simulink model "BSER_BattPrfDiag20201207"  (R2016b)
settings: Solver=FixedStepDiscrete  StartTime=0.0  StopTime=10.0  FixedStep=0.02  RelTol=1e-3  EnableMultiTasking=on
undefined symbols (not defined in the file or in its folder): bin2dec, BSER_cntBattOCMinDiag_C, BSER_cntBattPrfDiag_CW, BSER_cntChrgOCNpl_C, BSER_cntDisChOCNpl_C, BSER_cntPwrConvertConst_C, BSER_iChrgCurrErr_C, BSER_iChrgCurrOk_C, BSER_iDisChCurrErr_C, BSER_iDisChCurrOk_C, BSER_iLonChrgCurrErr_C, BSER_iLonChrgCurrOk_C, BSER_iLonDisChCurrErr_C, BSER_iLonDisChCurrOk_C, BSER_iShrtChrgCurrErr_C, BSER_iShrtChrgCurrOk_C, BSER_iShrtDisChCurrErr_C, BSER_iShrtDisChCurrOk_C, BSER_iSumLonChrgCurrReq_C, BSER_iSumLonDisChCurrReq_C, BSER_iSumShrtChrgCurrReq_C, BSER_iSumShrtDisChCurrReq_C, BSER_rLonChrgCurrHeal_C, BSER_rLonChrgCurrHi_C, BSER_rLonDisChCurrHeal_C, BSER_rLonDisChCurrHi_C, BSER_rShrtChrgCurrHeal_C, BSER_rShrtChrgCurrHi_C, BSER_rShrtDisChCurrHeal_C, BSER_rShrtDisChCurrHi_C, BSER_tiChrgCurrErr_C, BSER_tiChrgCurrOk_C, BSER_tiCurrConstPer_C, BSER_tiCurrPeakPer_C, BSER_tiDisChCurrErr_C, BSER_tiDisChCurrOk_C, BSER_uBattVoltConst_C
libraries: simulink x68
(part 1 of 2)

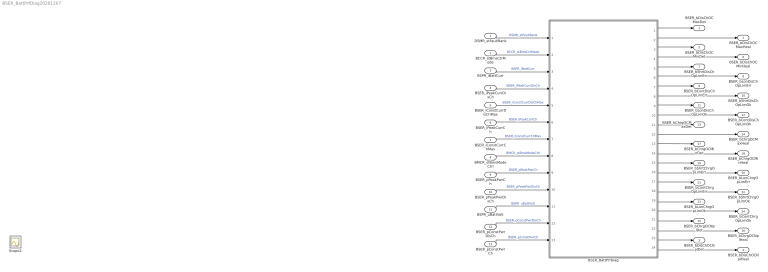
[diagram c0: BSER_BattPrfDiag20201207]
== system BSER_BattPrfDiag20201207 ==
  DSMR_stFaultRank : Inport
  BCCR_stBmsCtrMode : Inport  Port=2
  BSPR_iBattCurr : Inport  Port=3
  BSER_iPeakCurrDisCh : Inport  Port=4
  BSER_iConstCurrDisChMax : Inport  Port=5
  BSER_iPeakCurrCh : Inport  Port=6
  BSER_iConstCurrChMax : Inport  Port=7
  BMCR_stBmsModeCtrl : Inport  Port=8
  BSER_pPeakPwrCh : Inport  Port=9
  BSER_pPeakPwrDisCh : Inport  Port=10
  BSPR_uBattVolt : Inport  Port=11
  BSER_pConstPwrDisCh : Inport  Port=12
  BSER_pConstPwrCh : Inport  Port=13
  BSER_BattPrfDiag : Subsystem
  BSER_bDisChOCMaxDet : Outport
  BSER_bDisChOCMaxHeal : Outport  Port=2
  BSER_bDisChOCNplDet : Outport  Port=3
  BSER_bDisChOCNplHeal : Outport  Port=4
  BSER_bDisChOCMinDet : Outport  Port=5
  BSER_bDisChOCMinHeal : Outport  Port=6
  BSER_bShrtDisChOpLimErr : Outport  Port=7
  BSER_bLonDisChOpLimErr : Outport  Port=8
  BSER_bContDisChOpLimErr : Outport  Port=9
  BSER_bShrtDisChOpLimOk : Outport  Port=10
  BSER_bLonDisChOpLimOk : Outport  Port=11
  BSER_bContDisChOpLimOk : Outport  Port=12
  BSER_bChrgOCMaxDet : Outport  Port=13
  BSER_bChrgOCMaxHeal : Outport  Port=14
  BSER_bChrgOCNplDet : Outport  Port=15
  BSER_bChrgOCNplHeal : Outport  Port=16
  BSER_bChrgOCMinDet : Outport  Port=17
  BSER_bChrgOCMinHeal : Outport  Port=18
  BSER_bShrtChrgOpLimErr : Outport  Port=19
  BSER_bLonChrgOpLimErr : Outport  Port=20
  BSER_bContChrgOpLimErr : Outport  Port=21
  BSER_bShrtChrgOpLimOk : Outport  Port=22
  BSER_bLonChrgOpLimOk : Outport  Port=23
  BSER_bContChrgOpLimOk : Outport  Port=24
  Scope2 : Scope
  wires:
  DSMR_stFaultRank/1 -> BSER_BattPrfDiag/1(DSMR_stFaultRank)  "DSMR_stFaultRank"
  BCCR_stBmsCtrMode/1 -> BSER_BattPrfDiag/2(BCCR_stBmsCtrMode)  "BCCR_stBmsCtrMode"
  BSPR_iBattCurr/1 -> BSER_BattPrfDiag/3(BSPR_iBattCurr)  "BSPR_iBattCurr"
  BSER_iPeakCurrDisCh/1 -> BSER_BattPrfDiag/4(BSER_iPeakCurrDisCh)  "BSER_iPeakCurrDisCh"
  BSER_iConstCurrDisChMax/1 -> BSER_BattPrfDiag/5(BSER_iConstCurrDisChMax)  "BSER_iConstCurrDisChMax"
  BSER_iPeakCurrCh/1 -> BSER_BattPrfDiag/6(BSER_iPeakCurrCh)  "BSER_iPeakCurrCh"
  BSER_iConstCurrChMax/1 -> BSER_BattPrfDiag/7(BSER_iConstCurrChMax)  "BSER_iConstCurrChMax"
  BSER_BattPrfDiag/1(BSER_bDisChOCMaxDet) -> BSER_bDisChOCMaxDet/1
  BSER_BattPrfDiag/2(BSER_bDisChOCMaxHeal) -> BSER_bDisChOCMaxHeal/1
  BSER_BattPrfDiag/3(BSER_bDisChOCMinDet) -> BSER_bDisChOCMinDet/1
  BSER_BattPrfDiag/4(BSER_bDisChOCMinHeal) -> BSER_bDisChOCMinHeal/1
  BSER_BattPrfDiag/5(BSER_bShrtDisChOpLimErr) -> BSER_bShrtDisChOpLimErr/1
  BSER_BattPrfDiag/6(BSER_bLonDisChOpLimErr) -> BSER_bLonDisChOpLimErr/1
  BSER_BattPrfDiag/7(BSER_bContDisChOpLimErr) -> BSER_bContDisChOpLimErr/1
  BSER_BattPrfDiag/8(BSER_bShrtDisChOpLimOk) -> BSER_bShrtDisChOpLimOk/1
  BSER_BattPrfDiag/9(BSER_bLonDisChOpLimOk) -> BSER_bLonDisChOpLimOk/1
  BSER_BattPrfDiag/10(BSER_bContDisChOpLimOk) -> BSER_bContDisChOpLimOk/1
  BSER_BattPrfDiag/11(BSER_bChrgOCMaxDet) -> BSER_bChrgOCMaxDet/1
  BSER_BattPrfDiag/12(BSER_bChrgOCMaxHeal) -> BSER_bChrgOCMaxHeal/1
  BSER_BattPrfDiag/13(BSER_bChrgOCMinDet) -> BSER_bChrgOCMinDet/1
  BSER_BattPrfDiag/14(BSER_bChrgOCMinHeal) -> BSER_bChrgOCMinHeal/1
  BSER_BattPrfDiag/15(BSER_bShrtChrgOpLimErr) -> BSER_bShrtChrgOpLimErr/1
  BSER_BattPrfDiag/16(BSER_bLonChrgOpLimErr) -> BSER_bLonChrgOpLimErr/1
  BSER_BattPrfDiag/17(BSER_bContChrgOpLimErr) -> BSER_bContChrgOpLimErr/1
  BSER_BattPrfDiag/18(BSER_bShrtChrgOpLimOk) -> BSER_bShrtChrgOpLimOk/1
  BSER_BattPrfDiag/19(BSER_bLonChrgOpLimOk) -> BSER_bLonChrgOpLimOk/1
  BSER_BattPrfDiag/20(BSER_bContChrgOpLimOk) -> BSER_bContChrgOpLimOk/1
  BSER_BattPrfDiag/23(BSER_bDisChOCNplDet) -> BSER_bDisChOCNplDet/1
  BSER_BattPrfDiag/24(BSER_bDisChOCNplHeal) -> BSER_bDisChOCNplHeal/1
  BSER_BattPrfDiag/21(BSER_bChrgOCNplDet) -> BSER_bChrgOCNplDet/1
  BSER_BattPrfDiag/22(BSER_bChrgOCNplHeal) -> BSER_bChrgOCNplHeal/1
  BMCR_stBmsModeCtrl/1 -> BSER_BattPrfDiag/8(BMCR_stBmsModeCtrl)  "BMCR_stBmsModeCtrl"
  BSER_pPeakPwrDisCh/1 -> BSER_BattPrfDiag/10(BSER_pPeakPwrDisCh)  "BSER_pPeakPwrDisCh"
  BSER_pPeakPwrCh/1 -> BSER_BattPrfDiag/9(BSER_pPeakPwrCh)  "BSER_pPeakPwrCh"
  BSPR_uBattVolt/1 -> BSER_BattPrfDiag/11(BSPR_uBattVolt)  "BSPR_uBattVolt"
  BSER_pConstPwrCh/1 -> BSER_BattPrfDiag/13(BSER_pConstPwrCh)  "BSER_pConstPwrCh"
  BSER_pConstPwrDisCh/1 -> BSER_BattPrfDiag/12(BSER_pConstPwrDisCh)  "BSER_pConstPwrDisCh"

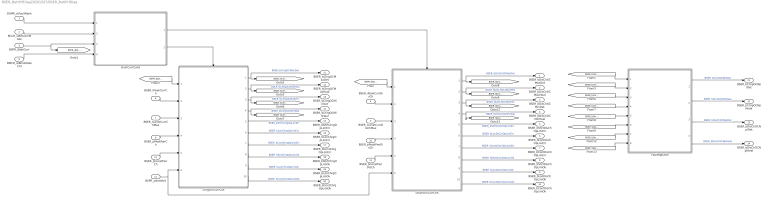
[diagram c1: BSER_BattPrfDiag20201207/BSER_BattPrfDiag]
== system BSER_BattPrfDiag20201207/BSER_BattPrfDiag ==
  DSMR_stFaultRank : Inport
  BCCR_stBmsCtrMode : Inport  Port=2
  BSPR_iBattCurr : Inport  Port=3
  BSER_iPeakCurrDisCh : Inport  Port=4
  BSER_iConstCurrDisChMax : Inport  Port=5
  BSER_iPeakCurrCh : Inport  Port=6
  BSER_iConstCurrChMax : Inport  Port=7
  BMCR_stBmsModeCtrl : Inport  Port=8
  BSER_pPeakPwrCh : Inport  Port=9
  BSER_pPeakPwrDisCh : Inport  Port=10
  BSPR_uBattVolt : Inport  Port=11
  BSER_pConstPwrDisCh : Inport  Port=12
  BSER_pConstPwrCh : Inport  Port=13
  ChrgOvrCurrChk : Subsystem
  DischOvrCurrChk : Subsystem
  FaultRptDsm : Subsystem
  OverCurrCond : Subsystem
  BSER_bDisChOCMaxDet : Outport
  BSER_bDisChOCMaxHeal : Outport  Port=2
  BSER_bDisChOCMinDet : Outport  Port=3
  BSER_bDisChOCMinHeal : Outport  Port=4
  BSER_bShrtDisChOpLimErr : Outport  Port=5
  BSER_bLonDisChOpLimErr : Outport  Port=6
  BSER_bContDisChOpLimErr : Outport  Port=7
  BSER_bShrtDisChOpLimOk : Outport  Port=8
  BSER_bLonDisChOpLimOk : Outport  Port=9
  BSER_bContDisChOpLimOk : Outport  Port=10
  BSER_bChrgOCMaxDet : Outport  Port=11
  BSER_bChrgOCMaxHeal : Outport  Port=12
  BSER_bChrgOCMinDet : Outport  Port=13
  BSER_bChrgOCMinHeal : Outport  Port=14
  BSER_bShrtChrgOpLimErr : Outport  Port=15
  BSER_bLonChrgOpLimErr : Outport  Port=16
  BSER_bContChrgOpLimErr : Outport  Port=17
  BSER_bShrtChrgOpLimOk : Outport  Port=18
  BSER_bLonChrgOpLimOk : Outport  Port=19
  BSER_bContChrgOpLimOk : Outport  Port=20
  BSER_bChrgOCNplDet : Outport  Port=21
  BSER_bChrgOCNplHeal : Outport  Port=22
  BSER_bDisChOCNplDet : Outport  Port=23
  BSER_bDisChOCNplHeal : Outport  Port=24
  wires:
  ChrgOvrCurrChk/10(BSER_bContChrgOpLimOk) -> BSER_bContChrgOpLimOk/1  "BSER_bContChrgOpLimOk"
  ChrgOvrCurrChk/9(BSER_bLonChrgOpLimOk) -> BSER_bLonChrgOpLimOk/1  "BSER_bLonChrgOpLimOk"
  ChrgOvrCurrChk/8(BSER_bShrtChrgOpLimOk) -> BSER_bShrtChrgOpLimOk/1  "BSER_bShrtChrgOpLimOk"
  ChrgOvrCurrChk/7(BSER_bContChrgOpLimErr) -> BSER_bContChrgOpLimErr/1  "BSER_bContChrgOpLimErr"
  ChrgOvrCurrChk/3(BSER_bChrgOCMinDet) -> [BSER_bChrgOCMinDet], BSER_bChrgOCMinDet/1  "BSER_bChrgOCMinDet"
  ChrgOvrCurrChk/6(BSER_bLonChrgOpLimErr) -> BSER_bLonChrgOpLimErr/1  "BSER_bLonChrgOpLimErr"
  ChrgOvrCurrChk/4(BSER_bChrgOCMinHeal) -> [BSER_bChrgOCMinHeal], BSER_bChrgOCMinHeal/1  "BSER_bChrgOCMinHeal"
  OverCurrCond/1(BSER_flgDisChOvrCurrCond) -> DischOvrCurrChk/Enable
  DischOvrCurrChk/8(BSER_bShrtDisChOpLimOk) -> BSER_bShrtDisChOpLimOk/1  "BSER_bShrtDisChOpLimOk"
  BSER_iPeakCurrCh/1 -> ChrgOvrCurrChk/2(BSER_iPeakCurrCh)
  [BSPR_iBattCurr] -> ChrgOvrCurrChk/1(BSPR_iBattCurr)
  DischOvrCurrChk/3(BSER_bDisChOCMinDet) -> BSER_bDisChOCMinDet/1, [BSER_bDisChOCMinDet]  "BSER_bDisChOCMinDet"
  OverCurrCond/2(BSER_flgChrgOvrCurrCond) -> ChrgOvrCurrChk/Enable
  [BSPR_iBattCurr] -> DischOvrCurrChk/1(BSPR_iBattCurr)
  DSMR_stFaultRank/1 -> OverCurrCond/1(DSMR_stFaultRank)
  ChrgOvrCurrChk/1(BSER_bChrgOCMaxDet) -> [BSER_bChrgOCMaxDet], BSER_bChrgOCMaxDet/1  "BSER_bChrgOCMaxDet"
  ChrgOvrCurrChk/2(BSER_bChrgOCMaxHeal) -> [BSER_bChrgOCMaxHeal], BSER_bChrgOCMaxHeal/1  "BSER_bChrgOCMaxHeal"
  DischOvrCurrChk/10(BSER_bContDisChOpLimOk) -> BSER_bContDisChOpLimOk/1  "BSER_bContDisChOpLimOk"
  DischOvrCurrChk/9(BSER_bLonDisChOpLimOk) -> BSER_bLonDisChOpLimOk/1  "BSER_bLonDisChOpLimOk"
  DischOvrCurrChk/7(BSER_bContDisChOpLimErr) -> BSER_bContDisChOpLimErr/1  "BSER_bContDisChOpLimErr"
  DischOvrCurrChk/5(BSER_bShrtDisChOpLimErr) -> BSER_bShrtDisChOpLimErr/1  "BSER_bShrtDisChOpLimErr"
  DischOvrCurrChk/6(BSER_bLonDisChOpLimErr) -> BSER_bLonDisChOpLimErr/1  "BSER_bLonDisChOpLimErr"
  BSER_iConstCurrChMax/1 -> ChrgOvrCurrChk/3(BSER_iConstCurrChMax)
  BCCR_stBmsCtrMode/1 -> OverCurrCond/2(BCCR_stBmsCtrMode)
  DischOvrCurrChk/1(BSER_bDisChOCMaxDet) -> [BSER_bDisChOCMaxDet], BSER_bDisChOCMaxDet/1  "BSER_bDisChOCMaxDet"
  DischOvrCurrChk/2(BSER_bDisChOCMaxHeal) -> [BSER_bDisChOCMaxHeal], BSER_bDisChOCMaxHeal/1  "BSER_bDisChOCMaxHeal"
  BSPR_iBattCurr/1 -> [BSPR_iBattCurr], OverCurrCond/3(BSPR_iBattCurr)
  BSER_iConstCurrDisChMax/1 -> DischOvrCurrChk/3(BSER_iConstCurrDisChMax)
  BSER_iPeakCurrDisCh/1 -> DischOvrCurrChk/2(BSER_iPeakCurrDisCh)
  ChrgOvrCurrChk/5(BSER_bShrtChrgOpLimErr) -> BSER_bShrtChrgOpLimErr/1  "BSER_bShrtChrgOpLimErr"
  [BSER_bDisChOCMinDet] -> FaultRptDsm/7(BSER_bDisChOCMinDet)
  [BSER_bDisChOCMinHeal] -> FaultRptDsm/8(BSER_bDisChOCMinHeal)
  [BSER_bDisChOCMaxHeal] -> FaultRptDsm/6(BSER_bDisChOCMaxHeal)
  [BSER_bDisChOCMaxDet] -> FaultRptDsm/5(BSER_bDisChOCMaxDet)
  [BSER_bChrgOCMaxHeal] -> FaultRptDsm/2(BSER_bChrgOCMaxHeal)
  [BSER_bChrgOCMaxDet] -> FaultRptDsm/1(BSER_bChrgOCMaxDet)
  [BSER_bChrgOCMinHeal] -> FaultRptDsm/4(BSER_bChrgOCMinHeal)
  [BSER_bChrgOCMinDet] -> FaultRptDsm/3(BSER_bChrgOCMinDet)
  DischOvrCurrChk/4(BSER_bDisChOCMinHeal) -> [BSER_bDisChOCMinHeal], BSER_bDisChOCMinHeal/1  "BSER_bDisChOCMinHeal"
  FaultRptDsm/1(BSER_bChrgOCNplDet) -> BSER_bChrgOCNplDet/1  "BSER_bChrgOCNplDet"
  FaultRptDsm/2(BSER_bChrgOCNplHeal) -> BSER_bChrgOCNplHeal/1  "BSER_bChrgOCNplHeal"
  FaultRptDsm/3(BSER_bDisChOCNplDet) -> BSER_bDisChOCNplDet/1  "BSER_bDisChOCNplDet"
  FaultRptDsm/4(BSER_bDisChOCNplHeal) -> BSER_bDisChOCNplHeal/1  "BSER_bDisChOCNplHeal"
  BMCR_stBmsModeCtrl/1 -> OverCurrCond/4(BMCR_stBmsModeCtrl)
  BSER_pPeakPwrCh/1 -> ChrgOvrCurrChk/4(BSER_pPeakPwrCh)
  BSER_pPeakPwrDisCh/1 -> DischOvrCurrChk/4(BSER_pPeakPwrDisCh)
  BSPR_uBattVolt/1 -> ChrgOvrCurrChk/6(BSPR_uBattVolt), DischOvrCurrChk/6(BSPR_uBattVolt)
  BSER_pConstPwrCh/1 -> ChrgOvrCurrChk/5(BSER_pConstPwrCh)
  BSER_pConstPwrDisCh/1 -> DischOvrCurrChk/5(BSER_pConstPwrDisCh)

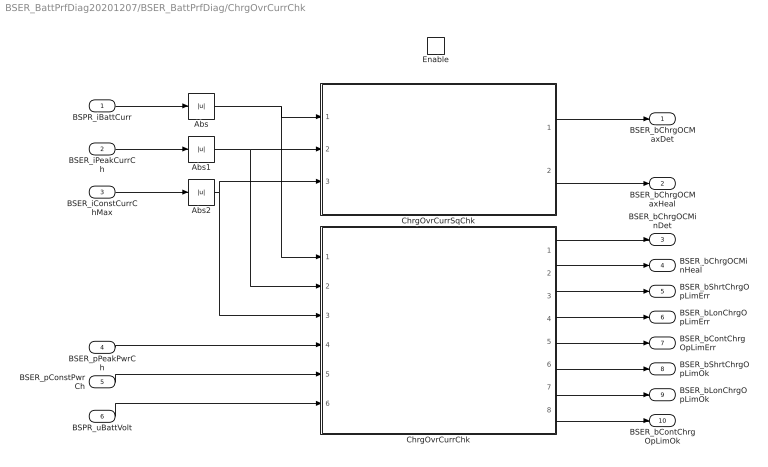
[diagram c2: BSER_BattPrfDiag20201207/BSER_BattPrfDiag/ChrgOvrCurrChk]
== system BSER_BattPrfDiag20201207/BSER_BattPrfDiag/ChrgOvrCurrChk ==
  BSPR_iBattCurr : Inport
  BSER_iPeakCurrCh : Inport  Port=2
  BSER_iConstCurrChMax : Inport  Port=3
  BSER_pPeakPwrCh : Inport  Port=4
  BSER_pConstPwrCh : Inport  Port=5
  BSPR_uBattVolt : Inport  Port=6
  Enable : EnablePort
  Abs : Abs
  Abs1 : Abs
  Abs2 : Abs
  ChrgOvrCurrChk : Subsystem
  ChrgOvrCurrSqChk : Subsystem
  BSER_bChrgOCMaxDet : Outport  InitialOutput=[0]
  BSER_bChrgOCMaxHeal : Outport  Port=2  InitialOutput=[0]
  BSER_bChrgOCMinDet : Outport  Port=3
  BSER_bChrgOCMinHeal : Outport  Port=4
  BSER_bShrtChrgOpLimErr : Outport  Port=5
  BSER_bLonChrgOpLimErr : Outport  Port=6
  BSER_bContChrgOpLimErr : Outport  Port=7
  BSER_bShrtChrgOpLimOk : Outport  Port=8
  BSER_bLonChrgOpLimOk : Outport  Port=9
  BSER_bContChrgOpLimOk : Outport  Port=10
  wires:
  ChrgOvrCurrChk/2(BSER_bChrgOCMinHeal) -> BSER_bChrgOCMinHeal/1
  ChrgOvrCurrSqChk/2(BSER_bChrgOCMaxHeal) -> BSER_bChrgOCMaxHeal/1
  ChrgOvrCurrSqChk/1(BSER_bChrgOCMaxDet) -> BSER_bChrgOCMaxDet/1
  ChrgOvrCurrChk/1(BSER_bChrgOCMinDet) -> BSER_bChrgOCMinDet/1
  BSPR_iBattCurr/1 -> Abs/1
  BSER_iConstCurrChMax/1 -> Abs2/1
  BSER_iPeakCurrCh/1 -> Abs1/1
  Abs/1 -> ChrgOvrCurrChk/1(BSPR_iCurr), ChrgOvrCurrSqChk/1(BSPR_iBattCurr)
  Abs1/1 -> ChrgOvrCurrChk/2(BSER_iPeakCurrCh), ChrgOvrCurrSqChk/2(BSER_iChgCurrShrtLim)
  Abs2/1 -> ChrgOvrCurrSqChk/3(BSER_iChgCurrLonLim), ChrgOvrCurrChk/3(BSER_iConstCurrChMax)
  ChrgOvrCurrChk/3(BSER_bShrtChrgOpLimErr) -> BSER_bShrtChrgOpLimErr/1
  ChrgOvrCurrChk/4(BSER_bLonChrgOpLimErr) -> BSER_bLonChrgOpLimErr/1
  ChrgOvrCurrChk/5(BSER_bContChrgOpLimErr) -> BSER_bContChrgOpLimErr/1
  ChrgOvrCurrChk/6(BSER_bShrtChrgOpLimOk) -> BSER_bShrtChrgOpLimOk/1
  ChrgOvrCurrChk/7(BSER_bLonChrgOpLimOk) -> BSER_bLonChrgOpLimOk/1
  ChrgOvrCurrChk/8(BSER_bContChrgOpLimOk) -> BSER_bContChrgOpLimOk/1
  BSER_pPeakPwrCh/1 -> ChrgOvrCurrChk/4(BSER_pPeakPwrCh)
  BSPR_uBattVolt/1 -> ChrgOvrCurrChk/6(BSPR_uBattVolt)
  BSER_pConstPwrCh/1 -> ChrgOvrCurrChk/5(BSER_pConstPwrCh)

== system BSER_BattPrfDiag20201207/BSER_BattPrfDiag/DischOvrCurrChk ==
  BSPR_iBattCurr : Inport
  BSER_iPeakCurrDisCh : Inport  Port=2
  BSER_iConstCurrDisChMax : Inport  Port=3
  BSER_pPeakPwrDisCh : Inport  Port=4
  BSER_pConstPwrDisCh : Inport  Port=5
  BSPR_uBattVolt : Inport  Port=6
  Enable : EnablePort
  DischOvrCurrChk : Subsystem
  DischOvrCurrSqChk : Subsystem
  BSER_bDisChOCMaxDet : Outport  InitialOutput=[0]
  BSER_bDisChOCMaxHeal : Outport  Port=2  InitialOutput=[0]
  BSER_bDisChOCMinDet : Outport  Port=3
  BSER_bDisChOCMinHeal : Outport  Port=4
  BSER_bShrtDisChOpLimErr : Outport  Port=5
  BSER_bLonDisChOpLimErr : Outport  Port=6
  BSER_bContDisChOpLimErr : Outport  Port=7
  BSER_bShrtDisChOpLimOk : Outport  Port=8
  BSER_bLonDisChOpLimOk : Outport  Port=9
  BSER_bContDisChOpLimOk : Outport  Port=10
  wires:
  BSER_iPeakCurrDisCh/1 -> DischOvrCurrChk/2(BSER_iPeakCurrDisCh), DischOvrCurrSqChk/2(BSER_iDisChCurrShrtLim)
  BSER_iConstCurrDisChMax/1 -> DischOvrCurrChk/3(BSER_iConstCurrDisChMax), DischOvrCurrSqChk/3(BSER_iDisChCurrLonLim)
  BSPR_iBattCurr/1 -> DischOvrCurrChk/1(BSPR_iCurr), DischOvrCurrSqChk/1(BSPR_iBattCurr)
  DischOvrCurrChk/1(BSER_bDisChOCMinDet) -> BSER_bDisChOCMinDet/1
  DischOvrCurrSqChk/1(BSER_bDisChOCMaxDet) -> BSER_bDisChOCMaxDet/1
  DischOvrCurrSqChk/2(BSER_bDisChOCErrHeal) -> BSER_bDisChOCMaxHeal/1
  DischOvrCurrChk/2(BSER_bDisChOCMinHeal) -> BSER_bDisChOCMinHeal/1
  DischOvrCurrChk/5(BSER_bContDisChOpLimErr) -> BSER_bContDisChOpLimErr/1
  DischOvrCurrChk/4(BSER_bLonDisChOpLimErr) -> BSER_bLonDisChOpLimErr/1
  DischOvrCurrChk/3(BSER_bShrtDisChOpLimErr) -> BSER_bShrtDisChOpLimErr/1
  DischOvrCurrChk/8(BSER_bContDisChOpLimOk) -> BSER_bContDisChOpLimOk/1
  DischOvrCurrChk/7(BSER_bLonDisChOpLimOk) -> BSER_bLonDisChOpLimOk/1
  DischOvrCurrChk/6(BSER_bShrtDisChOpLimOk) -> BSER_bShrtDisChOpLimOk/1
  BSER_pPeakPwrDisCh/1 -> DischOvrCurrChk/4(BSER_pPeakPwrDisCh)
  BSER_pConstPwrDisCh/1 -> DischOvrCurrChk/5(BSER_pConstPwrDisCh)
  BSPR_uBattVolt/1 -> DischOvrCurrChk/6(BSPR_uBattVolt)

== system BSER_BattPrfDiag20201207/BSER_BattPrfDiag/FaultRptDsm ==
  BSER_bChrgOCMaxDet : Inport
  BSER_bChrgOCMaxHeal : Inport  Port=2
  BSER_bChrgOCMinDet : Inport  Port=3
  BSER_bChrgOCMinHeal : Inport  Port=4
  BSER_bDisChOCMaxDet : Inport  Port=5
  BSER_bDisChOCMaxHeal : Inport  Port=6
  BSER_bDisChOCMinDet : Inport  Port=7
  BSER_bDisChOCMinHeal : Inport  Port=8
  ChrgRptDsm : Subsystem
  DisChrgRptDsm : Subsystem
  BSER_bChrgOCNplDet : Outport
  BSER_bChrgOCNplHeal : Outport  Port=2
  BSER_bDisChOCNplDet : Outport  Port=3
  BSER_bDisChOCNplHeal : Outport  Port=4
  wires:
  BSER_bChrgOCMaxDet/1 -> ChrgRptDsm/1(BSER_bChrgOCMaxDet)
  BSER_bChrgOCMaxHeal/1 -> ChrgRptDsm/2(BSER_bChrgOCMaxHeal)
  BSER_bChrgOCMinDet/1 -> ChrgRptDsm/3(BSER_bChrgOCMinDet)
  BSER_bChrgOCMinHeal/1 -> ChrgRptDsm/4(BSER_bChrgOCMinHeal)
  BSER_bDisChOCMaxDet/1 -> DisChrgRptDsm/1(BSER_bDisChOCMaxDet)
  BSER_bDisChOCMaxHeal/1 -> DisChrgRptDsm/2(BSER_bDisChOCMaxHeal)
  BSER_bDisChOCMinDet/1 -> DisChrgRptDsm/3(BSER_bDisChOCMinDet)
  BSER_bDisChOCMinHeal/1 -> DisChrgRptDsm/4(BSER_bDisChOCMinHeal)
  ChrgRptDsm/1(BSER_bChrgOCNplDet) -> BSER_bChrgOCNplDet/1
  ChrgRptDsm/2(BSER_bChrgOCNplHeal) -> BSER_bChrgOCNplHeal/1
  DisChrgRptDsm/1(BSER_bDisChOCNplDet) -> BSER_bDisChOCNplDet/1
  DisChrgRptDsm/2(BSER_bDisChOCNplHeal) -> BSER_bDisChOCNplHeal/1

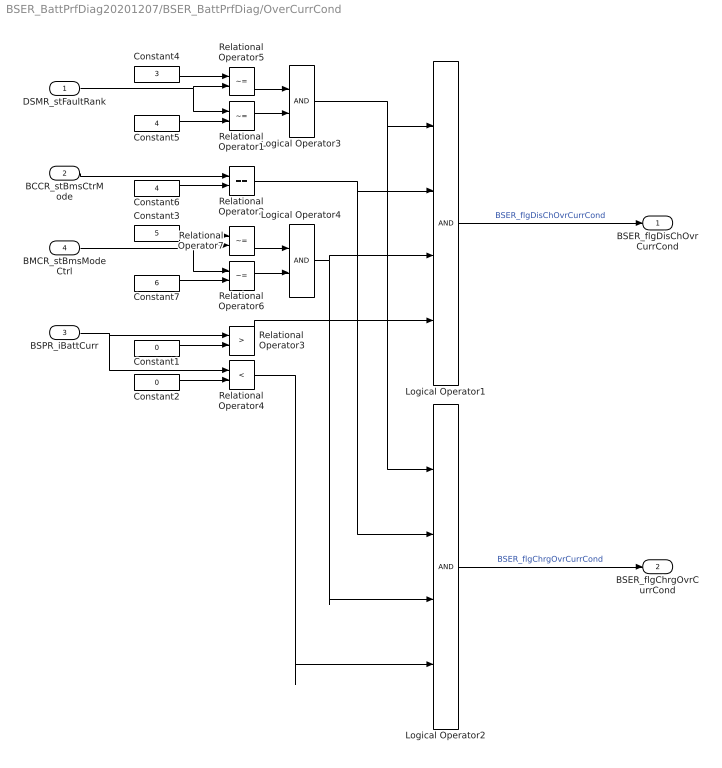
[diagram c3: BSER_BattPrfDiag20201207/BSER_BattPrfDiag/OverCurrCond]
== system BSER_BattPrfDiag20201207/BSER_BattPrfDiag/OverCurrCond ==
  DSMR_stFaultRank : Inport
  BCCR_stBmsCtrMode : Inport  Port=2
  BSPR_iBattCurr : Inport  Port=3
  BMCR_stBmsModeCtrl : Inport  Port=4
  Constant1 : Constant  Value=0  OutDataTypeStr=single
  Constant2 : Constant  Value=0  OutDataTypeStr=single
  Constant3 : Constant  Value=5  OutDataTypeStr=uint8
  Constant4 : Constant  Value=3  OutDataTypeStr=uint8
  Constant5 : Constant  Value=4  OutDataTypeStr=uint8
  Constant6 : Constant  Value=4  OutDataTypeStr=uint8
  Constant7 : Constant  Value=6  OutDataTypeStr=uint8
  Logical Operator1 : Logic  Inputs=4  AllPortsSameDT=off  OutDataTypeStr=boolean
  Logical Operator2 : Logic  Inputs=4  AllPortsSameDT=off  OutDataTypeStr=boolean
  Logical Operator3 : Logic  AllPortsSameDT=off  OutDataTypeStr=boolean
  Logical Operator4 : Logic  AllPortsSameDT=off  OutDataTypeStr=boolean
  Relational Operator{1,5..7} (4 alike) : RelationalOperator  Operator=~=  OutDataTypeStr=boolean  RndMeth=Simplest
  Relational Operator2 : RelationalOperator  Operator===  OutDataTypeStr=boolean  RndMeth=Simplest
  Relational Operator3 : RelationalOperator  Operator=>  OutDataTypeStr=boolean  RndMeth=Simplest
  Relational Operator4 : RelationalOperator  Operator=<  OutDataTypeStr=boolean  RndMeth=Simplest
  BSER_flgDisChOvrCurrCond : Outport
  BSER_flgChrgOvrCurrCond : Outport  Port=2
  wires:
  Logical Operator3/1 -> Logical Operator2/1, Logical Operator1/1
  Relational Operator5/1 -> Logical Operator3/1
  BCCR_stBmsCtrMode/1 -> Relational Operator2/1
  Constant4/1 -> Relational Operator5/1
  DSMR_stFaultRank/1 -> Relational Operator1/1, Relational Operator5/2
  Relational Operator1/1 -> Logical Operator3/2
  Constant5/1 -> Relational Operator1/2
  Constant6/1 -> Relational Operator2/2
  Relational Operator2/1 -> Logical Operator2/2, Logical Operator1/2
  Logical Operator1/1 -> BSER_flgDisChOvrCurrCond/1  "BSER_flgDisChOvrCurrCond"
  Constant1/1 -> Relational Operator3/2
  BSPR_iBattCurr/1 -> Relational Operator4/1, Relational Operator3/1
  Logical Operator2/1 -> BSER_flgChrgOvrCurrCond/1  "BSER_flgChrgOvrCurrCond"
  Constant2/1 -> Relational Operator4/2
  Relational Operator4/1 -> Logical Operator2/4
  Relational Operator7/1 -> Logical Operator4/1
  Constant3/1 -> Relational Operator7/1
  BMCR_stBmsModeCtrl/1 -> Relational Operator6/1, Relational Operator7/2
  Relational Operator6/1 -> Logical Operator4/2
  Constant7/1 -> Relational Operator6/2
  Relational Operator3/1 -> Logical Operator1/4
  Logical Operator4/1 -> Logical Operator1/3, Logical Operator2/3

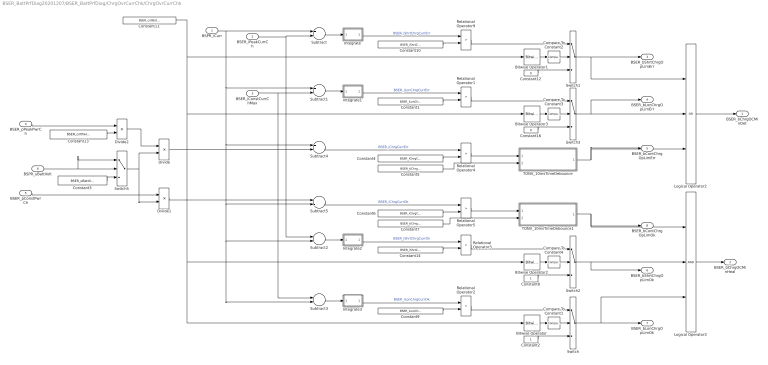
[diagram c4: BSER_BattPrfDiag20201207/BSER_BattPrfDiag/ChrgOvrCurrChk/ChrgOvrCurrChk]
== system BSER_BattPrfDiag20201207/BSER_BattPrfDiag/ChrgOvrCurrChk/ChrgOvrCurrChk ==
  BSPR_iCurr : Inport
  BSER_iPeakCurrCh : Inport  Port=2
  BSER_iConstCurrChMax : Inport  Port=3
  BSER_pPeakPwrCh : Inport  Port=4
  BSER_pConstPwrCh : Inport  Port=5
  BSPR_uBattVolt : Inport  Port=6
  Bitwise Operator : simulink/Logic and Bit Operations/Bitwise Operator  logicop=AND  UseBitMask=on  BitMask=bin2dec('00001000')  BitMaskRealWorld=Stored Integer
  Bitwise Operator1 : simulink/Logic and Bit Operations/Bitwise Operator  logicop=AND  UseBitMask=on  BitMask=bin2dec('00000100')  BitMaskRealWorld=Stored Integer
  Bitwise Operator2 : simulink/Logic and Bit Operations/Bitwise Operator  logicop=AND  UseBitMask=on  BitMask=bin2dec('00000100')  BitMaskRealWorld=Stored Integer
  Bitwise Operator3 : simulink/Logic and Bit Operations/Bitwise Operator  logicop=AND  UseBitMask=on  BitMask=bin2dec('00001000')  BitMaskRealWorld=Stored Integer
  Compare To Constant1 : simulink/Logic and Bit Operations/Compare To Constant  relop===  const=8  OutDataTypeStr=boolean
  Compare To Constant2 : simulink/Logic and Bit Operations/Compare To Constant  relop===  const=4  OutDataTypeStr=boolean
  Compare To Constant3 : simulink/Logic and Bit Operations/Compare To Constant  relop===  const=8  OutDataTypeStr=boolean
  Compare To Constant4 : simulink/Logic and Bit Operations/Compare To Constant  relop===  const=4  OutDataTypeStr=boolean
  Constant1 : Constant  Value=BSER_iLonChrgCurrErr_C
  Constant10 : Constant  Value=BSER_iShrtChrgCurrErr_C
  Constant11 : Constant  Value=BSER_cntBattOCMinDiag_C
  Constant12 : Constant  Value=0  OutDataTypeStr=boolean
  Constant13 : Constant  Value=BSER_cntPwrConvertConst_C
  Constant14 : Constant  Value=BSER_iShrtChrgCurrOk_C  OutDataTypeStr=single
  Constant16 : Constant  Value=0  OutDataTypeStr=boolean
  Constant2 : Constant  OutDataTypeStr=boolean
  Constant3 : Constant  Value=BSER_uBattVoltConst_C
  Constant4 : Constant  Value=BSER_iChrgCurrErr_C
  Constant5 : Constant  Value=BSER_tiChrgCurrErr_C
  Constant6 : Constant  Value=BSER_iChrgCurrOk_C
  Constant7 : Constant  Value=BSER_tiChrgCurrOk_C
  Constant8 : Constant  OutDataTypeStr=boolean
  Constant9 : Constant  Value=BSER_iLonChrgCurrOk_C  OutDataTypeStr=single
  Divide : Product  Inputs=*/
  Divide1 : Product  Inputs=*/
  Divide2 : Product  Inputs=**
  Integrate : Subsystem
  Integrate1 : Subsystem
  Integrate2 : Subsystem
  Integrate3 : Subsystem
  Logical Operator2 : Logic  Operator=OR  Inputs=3  AllPortsSameDT=off  OutDataTypeStr=boolean
  Logical Operator3 : Logic  Inputs=3  AllPortsSameDT=off  OutDataTypeStr=boolean
  Relational Operator{1..5,9} (6 alike) : RelationalOperator  Operator=>  OutDataTypeStr=boolean  RndMeth=Simplest
  Subtract{,1..5} (6 alike) : Sum  Inputs=+-
  Switch{,1..3} (4 alike) : Switch  Criteria=u2 > Threshold
  Switch5 : Switch  Criteria=u2 ~= 0
  TONV_10msTimeDebounce : Subsystem  TreatAsAtomicUnit=on  RTWFcnName=TONV_10msTimeDebounce  RTWFileName=SrvLib
  TONV_10msTimeDebounce1 : Subsystem  TreatAsAtomicUnit=on  RTWFcnName=TONV_10msTimeDebounce  RTWFileName=SrvLib
  BSER_bChrgOCMinDet : Outport
  BSER_bChrgOCMinHeal : Outport  Port=2
  BSER_bShrtChrgOpLimErr : Outport  Port=3
  BSER_bLonChrgOpLimErr : Outport  Port=4
  BSER_bContChrgOpLimErr : Outport  Port=5
  BSER_bShrtChrgOpLimOk : Outport  Port=6
  BSER_bLonChrgOpLimOk : Outport  Port=7
  BSER_bContChrgOpLimOk : Outport  Port=8
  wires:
  Constant14/1 -> Relational Operator3/2
  Logical Operator3/1 -> BSER_bChrgOCMinHeal/1
  Switch/1 -> BSER_bLonChrgOpLimOk/1, Logical Operator3/3
  Subtract5/1 -> Relational Operator5/1  "BSER_iChrgCurrOk"
  Constant7/1 -> TONV_10msTimeDebounce1/2(T)
  Relational Operator5/1 -> TONV_10msTimeDebounce1/1(u)
  Constant6/1 -> Relational Operator5/2
  Subtract4/1 -> Relational Operator4/1  "BSER_iChrgCurrErr"
  Constant5/1 -> TONV_10msTimeDebounce/2(T)
  Relational Operator4/1 -> TONV_10msTimeDebounce/1(u)
  Constant4/1 -> Relational Operator4/2
  Subtract3/1 -> Integrate3/1(In)
  Subtract2/1 -> Integrate2/1(In)
  Integrate3/1(Out) -> Relational Operator2/1  "BSER_iLonChrgCurrOk"
  Integrate2/1(Out) -> Relational Operator3/1  "BSER_iShrtChrgCurrOk"
  Constant1/1 -> Relational Operator1/2
  Integrate1/1(Out) -> Relational Operator1/1  "BSER_iLonChrgCurrErr"
  Constant10/1 -> Relational Operator9/2
  Subtract/1 -> Integrate/1(In)
  Subtract1/1 -> Integrate1/1(In)
  BSER_iPeakCurrCh/1 -> Subtract/2, Subtract2/1
  BSPR_iCurr/1 -> Subtract/1, Subtract3/2, Subtract2/2, Subtract5/2, Subtract4/1, Subtract1/1
  Logical Operator2/1 -> BSER_bChrgOCMinDet/1
  Switch1/1 -> BSER_bShrtChrgOpLimErr/1, Logical Operator2/1
  Switch3/1 -> Logical Operator2/2, BSER_bLonChrgOpLimErr/1
  TONV_10msTimeDebounce/1(y) -> Logical Operator2/3, BSER_bContChrgOpLimErr/1
  TONV_10msTimeDebounce1/1(y) -> Logical Operator3/1, BSER_bContChrgOpLimOk/1
  Switch2/1 -> Logical Operator3/2, BSER_bShrtChrgOpLimOk/1
  BSER_iConstCurrChMax/1 -> Subtract1/2, Subtract3/1
  Constant11/1 -> Bitwise Operator/1, Bitwise Operator2/1, Bitwise Operator3/1, Bitwise Operator1/1
  Bitwise Operator/1 -> Compare To Constant1/1
  Constant12/1 -> Switch1/3
  Bitwise Operator1/1 -> Compare To Constant2/1
  Bitwise Operator2/1 -> Compare To Constant4/1
  Constant16/1 -> Switch3/3
  Bitwise Operator3/1 -> Compare To Constant3/1
  Compare To Constant2/1 -> Switch1/2
  Compare To Constant3/1 -> Switch3/2
  Compare To Constant1/1 -> Switch/2
  Compare To Constant4/1 -> Switch2/2
  Constant8/1 -> Switch2/3
  Constant2/1 -> Switch/3
  Integrate/1(Out) -> Relational Operator9/1  "BSER_iShrtChrgCurrErr"
  Relational Operator9/1 -> Switch1/1
  Relational Operator1/1 -> Switch3/1
  Relational Operator3/1 -> Switch2/1
  Constant9/1 -> Relational Operator2/2
  Relational Operator2/1 -> Switch/1
  BSPR_uBattVolt/1 -> Switch5/2, Switch5/1
  Constant3/1 -> Switch5/3
  BSER_pPeakPwrCh/1 -> Divide2/1
  BSER_pConstPwrCh/1 -> Divide1/1
  Switch5/1 -> Divide1/2, Divide/2
  Divide1/1 -> Subtract5/1
  Divide/1 -> Subtract4/2
  Divide2/1 -> Divide/1
  Constant13/1 -> Divide2/2

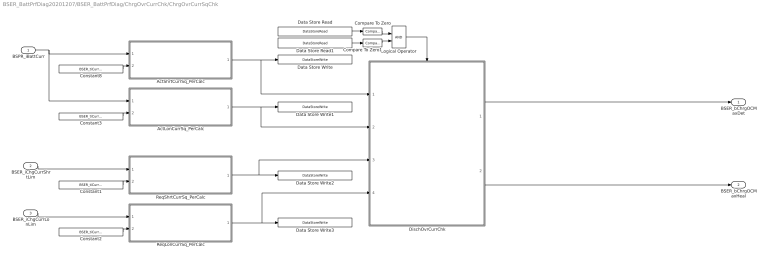
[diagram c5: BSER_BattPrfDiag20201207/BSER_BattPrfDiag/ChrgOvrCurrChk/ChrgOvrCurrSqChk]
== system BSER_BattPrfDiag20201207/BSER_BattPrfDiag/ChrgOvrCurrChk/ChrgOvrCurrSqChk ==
  BSPR_iBattCurr : Inport
  BSER_iChgCurrShrtLim : Inport  Port=2
  BSER_iChgCurrLonLim : Inport  Port=3
  ActLonCurrSq_PerCalc : Subsystem
  ActShrtCurrSq_PerCalc : Subsystem
  Compare To Zero : simulink/Logic and Bit Operations/Compare To Zero  relop=>  OutDataTypeStr=boolean
  Compare To Zero1 : simulink/Logic and Bit Operations/Compare To Zero  relop=>  OutDataTypeStr=boolean
  Constant1 : Constant  Value=BSER_tiCurrPeakPer_C
  Constant2 : Constant  Value=BSER_tiCurrConstPer_C
  Constant3 : Constant  Value=BSER_tiCurrConstPer_C
  Constant8 : Constant  Value=BSER_tiCurrPeakPer_C
  Data Store Read : DataStoreRead  DataStoreName=BSER_iSumShrtChrgCurrReq
  Data Store Read1 : DataStoreRead  DataStoreName=BSER_iSumLonChrgCurrReq
  Data Store Write : DataStoreWrite  DataStoreName=BSER_iSumShrtChrgCurrAct
  Data Store Write1 : DataStoreWrite  DataStoreName=BSER_iSumLonChrgCurrAct
  Data Store Write2 : DataStoreWrite  DataStoreName=BSER_iSumShrtChrgCurrReq
  Data Store Write3 : DataStoreWrite  DataStoreName=BSER_iSumLonChrgCurrReq
  DischOvrCurrChk : Subsystem
  Logical Operator : Logic  AllPortsSameDT=off  OutDataTypeStr=boolean
  ReqLonCurrSq_PerCalc : Subsystem
  ReqShrtCurrSq_PerCalc : Subsystem
  BSER_bChrgOCMaxDet : Outport
  BSER_bChrgOCMaxHeal : Outport  Port=2
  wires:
  BSPR_iBattCurr/1 -> ActLonCurrSq_PerCalc/1(BSPR_iCurr), ActShrtCurrSq_PerCalc/1(BSPR_iCurr)
  BSER_iChgCurrShrtLim/1 -> ReqShrtCurrSq_PerCalc/1(BSPR_iCurr)
  BSER_iChgCurrLonLim/1 -> ReqLonCurrSq_PerCalc/1(BSPR_iCurr)
  DischOvrCurrChk/2(BSER_bChrgOCMaxHeal) -> BSER_bChrgOCMaxHeal/1
  DischOvrCurrChk/1(BSER_bChrgOCMaxDet) -> BSER_bChrgOCMaxDet/1
  ActLonCurrSq_PerCalc/1(BSER_iCurrPerAcm) -> Data Store Write1/1, DischOvrCurrChk/2(BSER_iSumLonChrgCurrAct)
  ActShrtCurrSq_PerCalc/1(BSER_iCurrPerAcm) -> Data Store Write/1, DischOvrCurrChk/1(BSER_iSumShrtChrgCurrAct)
  Constant3/1 -> ActLonCurrSq_PerCalc/2(BSER_tiCurrConstPer_C)
  ReqLonCurrSq_PerCalc/1(BSER_iCurrPerAcm) -> Data Store Write3/1, DischOvrCurrChk/4(BSER_iSumLonChrgCurrReq)
  Constant1/1 -> ReqShrtCurrSq_PerCalc/2(BSER_tiCurrConstPer_C)
  Constant8/1 -> ActShrtCurrSq_PerCalc/2(BSER_tiCurrConstPer_C)
  ReqShrtCurrSq_PerCalc/1(BSER_iCurrPerAcm) -> Data Store Write2/1, DischOvrCurrChk/3(BSER_iSumShrtChrgCurrReq)
  Constant2/1 -> ReqLonCurrSq_PerCalc/2(BSER_tiCurrConstPer_C)
  Data Store Read/1 -> Compare To Zero/1
  Compare To Zero/1 -> Logical Operator/1
  Data Store Read1/1 -> Compare To Zero1/1
  Compare To Zero1/1 -> Logical Operator/2
  Logical Operator/1 -> DischOvrCurrChk/Enable

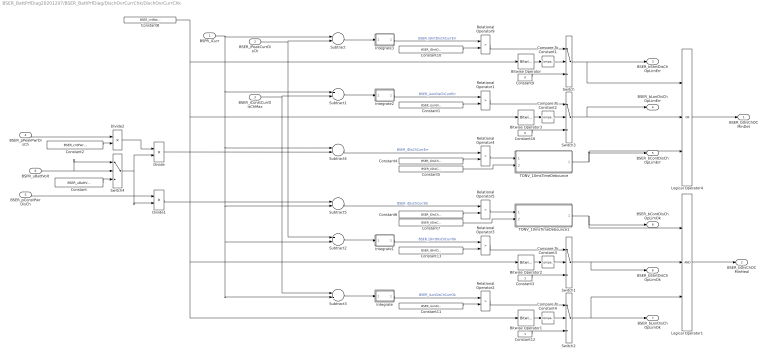
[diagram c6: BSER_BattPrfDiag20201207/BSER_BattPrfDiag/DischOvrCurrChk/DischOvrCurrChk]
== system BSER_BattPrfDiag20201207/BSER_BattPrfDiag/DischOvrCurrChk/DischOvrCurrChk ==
  BSPR_iCurr : Inport
  BSER_iPeakCurrDisCh : Inport  Port=2
  BSER_iConstCurrDisChMax : Inport  Port=3
  BSER_pPeakPwrDisCh : Inport  Port=4
  BSER_pConstPwrDisCh : Inport  Port=5
  BSPR_uBattVolt : Inport  Port=6
  Bitwise Operator : simulink/Logic and Bit Operations/Bitwise Operator  logicop=AND  UseBitMask=on  BitMask=bin2dec('00000001')  BitMaskRealWorld=Stored Integer
  Bitwise Operator1 : simulink/Logic and Bit Operations/Bitwise Operator  logicop=AND  UseBitMask=on  BitMask=bin2dec('00000010')  BitMaskRealWorld=Stored Integer
  Bitwise Operator2 : simulink/Logic and Bit Operations/Bitwise Operator  logicop=AND  UseBitMask=on  BitMask=bin2dec('00000001')  BitMaskRealWorld=Stored Integer
  Bitwise Operator3 : simulink/Logic and Bit Operations/Bitwise Operator  logicop=AND  UseBitMask=on  BitMask=bin2dec('00000010')  BitMaskRealWorld=Stored Integer
  Compare To Constant1 : simulink/Logic and Bit Operations/Compare To Constant  relop===  const=1  OutDataTypeStr=boolean
  Compare To Constant2 : simulink/Logic and Bit Operations/Compare To Constant  relop===  const=2  OutDataTypeStr=boolean
  Compare To Constant3 : simulink/Logic and Bit Operations/Compare To Constant  relop===  const=1  OutDataTypeStr=boolean
  Compare To Constant4 : simulink/Logic and Bit Operations/Compare To Constant  relop===  const=2  OutDataTypeStr=boolean
  Constant : Constant  Value=BSER_uBattVoltConst_C
  Constant1 : Constant  Value=BSER_iLonDisChCurrErr_C
  Constant10 : Constant  Value=BSER_iShrtDisChCurrErr_C
  Constant11 : Constant  Value=BSER_iLonDisChCurrOk_C  OutDataTypeStr=single
  Constant12 : Constant  OutDataTypeStr=boolean
  Constant13 : Constant  Value=BSER_iShrtDisChCurrOk_C  OutDataTypeStr=single
  Constant16 : Constant  Value=0  OutDataTypeStr=boolean
  Constant2 : Constant  Value=BSER_cntPwrConvertConst_C
  Constant3 : Constant  OutDataTypeStr=boolean
  Constant4 : Constant  Value=BSER_iDisChCurrErr_C
  Constant5 : Constant  Value=BSER_tiDisChCurrErr_C
  Constant6 : Constant  Value=BSER_iDisChCurrOk_C
  Constant7 : Constant  Value=BSER_tiDisChCurrOk_C
  Constant8 : Constant  Value=BSER_cntBattOCMinDiag_C
  Constant9 : Constant  Value=0  OutDataTypeStr=boolean
  Divide : Product  Inputs=*/
  Divide1 : Product  Inputs=*/
  Divide2 : Product  Inputs=**
  Integrate : Subsystem
  Integrate1 : Subsystem
  Integrate2 : Subsystem
  Integrate3 : Subsystem
  Logical Operator1 : Logic  Inputs=3  AllPortsSameDT=off  OutDataTypeStr=boolean
  Logical Operator4 : Logic  Operator=OR  Inputs=3  AllPortsSameDT=off  OutDataTypeStr=boolean
  Relational Operator{1..5,9} (6 alike) : RelationalOperator  Operator=>  OutDataTypeStr=boolean  RndMeth=Simplest
  Subtract{,1..5} (6 alike) : Sum  Inputs=+-
  Switch{,1..3} (4 alike) : Switch  Criteria=u2 > Threshold
  Switch4 : Switch  Criteria=u2 ~= 0
  TONV_10msTimeDebounce : Subsystem  TreatAsAtomicUnit=on  RTWFcnName=TONV_10msTimeDebounce  RTWFileName=SrvLib
  TONV_10msTimeDebounce1 : Subsystem  TreatAsAtomicUnit=on  RTWFcnName=TONV_10msTimeDebounce  RTWFileName=SrvLib
  BSER_bDisChOCMinDet : Outport
  BSER_bDisChOCMinHeal : Outport  Port=2
  BSER_bShrtDisChOpLimErr : Outport  Port=3
  BSER_bLonDisChOpLimErr : Outport  Port=4
  BSER_bContDisChOpLimErr : Outport  Port=5
  BSER_bShrtDisChOpLimOk : Outport  Port=6
  BSER_bLonDisChOpLimOk : Outport  Port=7
  BSER_bContDisChOpLimOk : Outport  Port=8
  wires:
  Logical Operator4/1 -> BSER_bDisChOCMinDet/1
  BSPR_iCurr/1 -> Subtract3/2, Subtract2/2, Subtract5/2, Subtract4/1, Subtract1/1, Subtract/1
  BSER_iConstCurrDisChMax/1 -> Subtract3/1, Subtract1/2
  Subtract1/1 -> Integrate2/1(In)
  Integrate3/1(Out) -> Relational Operator9/1  "BSER_iShrtDisChCurrErr"
  Constant10/1 -> Relational Operator9/2
  Integrate2/1(Out) -> Relational Operator1/1  "BSER_iLonDisChCurrErr"
  Constant1/1 -> Relational Operator1/2
  Constant11/1 -> Relational Operator2/2
  Integrate1/1(Out) -> Relational Operator3/1  "BSER_iShrtDisChCurrOk"
  Integrate/1(Out) -> Relational Operator2/1  "BSER_iLonDisChCurrOk"
  Subtract2/1 -> Integrate1/1(In)
  Subtract3/1 -> Integrate/1(In)
  Constant4/1 -> Relational Operator4/2
  Relational Operator4/1 -> TONV_10msTimeDebounce/1(u)
  Constant5/1 -> TONV_10msTimeDebounce/2(T)
  BSER_iPeakCurrDisCh/1 -> Subtract2/1, Subtract/2
  Subtract4/1 -> Relational Operator4/1  "BSER_iDisChCurrErr"
  Switch/1 -> Logical Operator4/1, BSER_bShrtDisChOpLimErr/1
  Switch3/1 -> BSER_bLonDisChOpLimErr/1, Logical Operator4/2
  TONV_10msTimeDebounce/1(y) -> BSER_bContDisChOpLimErr/1, Logical Operator4/3
  Constant6/1 -> Relational Operator5/2
  Relational Operator5/1 -> TONV_10msTimeDebounce1/1(u)
  Constant7/1 -> TONV_10msTimeDebounce1/2(T)
  Subtract5/1 -> Relational Operator5/1  "BSER_iDisChCurrOk"
  Logical Operator1/1 -> BSER_bDisChOCMinHeal/1
  Constant13/1 -> Relational Operator3/2
  TONV_10msTimeDebounce1/1(y) -> BSER_bContDisChOpLimOk/1, Logical Operator1/1
  Switch1/1 -> BSER_bShrtDisChOpLimOk/1, Logical Operator1/2
  Switch2/1 -> Logical Operator1/3, BSER_bLonDisChOpLimOk/1
  Subtract/1 -> Integrate3/1(In)
  Constant9/1 -> Switch/3
  Bitwise Operator/1 -> Compare To Constant1/1
  Bitwise Operator2/1 -> Compare To Constant3/1
  Constant8/1 -> Bitwise Operator3/1, Bitwise Operator1/1, Bitwise Operator2/1, Bitwise Operator/1
  Bitwise Operator1/1 -> Compare To Constant4/1
  Constant12/1 -> Switch2/3
  Bitwise Operator3/1 -> Compare To Constant2/1
  Constant16/1 -> Switch3/3
  Constant3/1 -> Switch1/3
  Compare To Constant1/1 -> Switch/2
  Compare To Constant2/1 -> Switch3/2
  Compare To Constant3/1 -> Switch1/2
  Compare To Constant4/1 -> Switch2/2
  Relational Operator9/1 -> Switch/1
  Relational Operator1/1 -> Switch3/1
  Relational Operator3/1 -> Switch1/1
  Relational Operator2/1 -> Switch2/1
  BSPR_uBattVolt/1 -> Switch4/2, Switch4/1
  Constant/1 -> Switch4/3
  Divide/1 -> Subtract4/2
  BSER_pConstPwrDisCh/1 -> Divide1/1
  Switch4/1 -> Divide1/2, Divide/2
  Divide1/1 -> Subtract5/1
  BSER_pPeakPwrDisCh/1 -> Divide2/1
  Divide2/1 -> Divide/1
  Constant2/1 -> Divide2/2

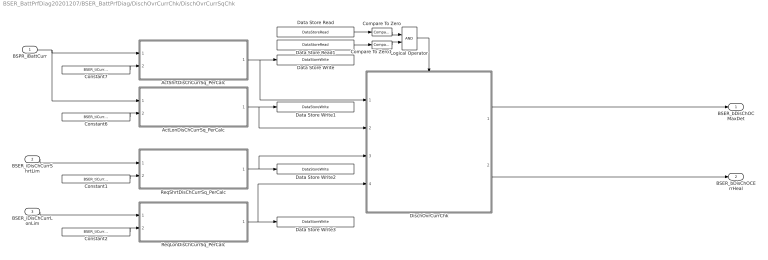
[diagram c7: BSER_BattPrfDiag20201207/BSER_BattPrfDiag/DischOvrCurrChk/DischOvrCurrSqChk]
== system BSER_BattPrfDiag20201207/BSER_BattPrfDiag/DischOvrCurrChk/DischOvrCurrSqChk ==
  BSPR_iBattCurr : Inport
  BSER_iDisChCurrShrtLim : Inport  Port=2
  BSER_iDisChCurrLonLim : Inport  Port=3
  ActLonDisChCurrSq_PerCalc : Subsystem
  ActShrtDisChCurrSq_PerCalc : Subsystem
  Compare To Zero : simulink/Logic and Bit Operations/Compare To Zero  relop=>  OutDataTypeStr=boolean
  Compare To Zero1 : simulink/Logic and Bit Operations/Compare To Zero  relop=>  OutDataTypeStr=boolean
  Constant1 : Constant  Value=BSER_tiCurrPeakPer_C
  Constant2 : Constant  Value=BSER_tiCurrConstPer_C
  Constant6 : Constant  Value=BSER_tiCurrConstPer_C
  Constant7 : Constant  Value=BSER_tiCurrPeakPer_C
  Data Store Read : DataStoreRead  DataStoreName=BSER_iSumShrtDisChCurrReq
  Data Store Read1 : DataStoreRead  DataStoreName=BSER_iSumLonDisChCurrReq
  Data Store Write : DataStoreWrite  DataStoreName=BSER_iSumShrtDisChCurrAct
  Data Store Write1 : DataStoreWrite  DataStoreName=BSER_iSumLonDisChCurrAct
  Data Store Write2 : DataStoreWrite  DataStoreName=BSER_iSumShrtDisChCurrReq
  Data Store Write3 : DataStoreWrite  DataStoreName=BSER_iSumLonDisChCurrReq
  DischOvrCurrChk : Subsystem
  Logical Operator : Logic  AllPortsSameDT=off  OutDataTypeStr=boolean
  ReqLonDisChCurrSq_PerCalc : Subsystem
  ReqShrtDisChCurrSq_PerCalc : Subsystem
  BSER_bDisChOCMaxDet : Outport
  BSER_bDisChOCErrHeal : Outport  Port=2
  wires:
  Constant2/1 -> ReqLonDisChCurrSq_PerCalc/2(BSER_tiCurrConstPer_C)
  ReqShrtDisChCurrSq_PerCalc/1(BSER_iCurrPerAcm) -> Data Store Write2/1, DischOvrCurrChk/3(BSER_iSumShrtDisChCurrReq)
  Constant7/1 -> ActShrtDisChCurrSq_PerCalc/2(BSER_tiCurrConstPer_C)
  Constant1/1 -> ReqShrtDisChCurrSq_PerCalc/2(BSER_tiCurrConstPer_C)
  ReqLonDisChCurrSq_PerCalc/1(BSER_iCurrPerAcm) -> Data Store Write3/1, DischOvrCurrChk/4(BSER_iSumLonDisChCurrReq)
  Constant6/1 -> ActLonDisChCurrSq_PerCalc/2(BSER_tiCurrConstPer_C)
  ActShrtDisChCurrSq_PerCalc/1(BSER_iCurrPerAcm) -> Data Store Write/1, DischOvrCurrChk/1(BSER_iSumShrtDisChCurrAct)
  ActLonDisChCurrSq_PerCalc/1(BSER_iCurrPerAcm) -> Data Store Write1/1, DischOvrCurrChk/2(BSER_iSumLonDisChCurrAct)
  DischOvrCurrChk/1(BSER_bDisChOCMaxDet) -> BSER_bDisChOCMaxDet/1
  DischOvrCurrChk/2(BSER_bDisChOCMaxHeal) -> BSER_bDisChOCErrHeal/1
  BSER_iDisChCurrLonLim/1 -> ReqLonDisChCurrSq_PerCalc/1(BSPR_iCurr)
  BSER_iDisChCurrShrtLim/1 -> ReqShrtDisChCurrSq_PerCalc/1(BSPR_iCurr)
  BSPR_iBattCurr/1 -> ActLonDisChCurrSq_PerCalc/1(BSPR_iCurr), ActShrtDisChCurrSq_PerCalc/1(BSPR_iCurr)
  Compare To Zero/1 -> Logical Operator/1
  Compare To Zero1/1 -> Logical Operator/2
  Logical Operator/1 -> DischOvrCurrChk/Enable
  Data Store Read/1 -> Compare To Zero/1
  Data Store Read1/1 -> Compare To Zero1/1

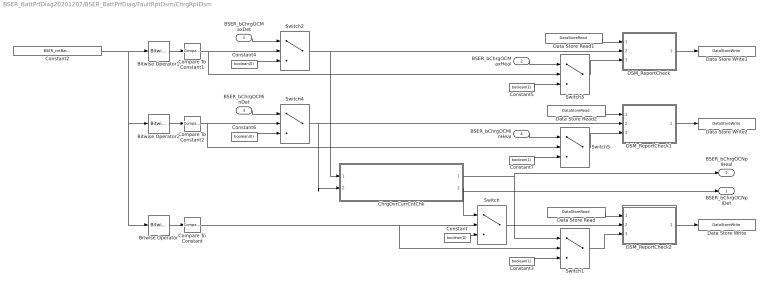
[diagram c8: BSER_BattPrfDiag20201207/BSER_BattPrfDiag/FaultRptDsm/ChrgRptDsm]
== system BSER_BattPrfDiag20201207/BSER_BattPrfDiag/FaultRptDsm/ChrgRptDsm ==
  BSER_bChrgOCMaxDet : Inport
  BSER_bChrgOCMaxHeal : Inport  Port=2
  BSER_bChrgOCMinDet : Inport  Port=3
  BSER_bChrgOCMinHeal : Inport  Port=4
  Bitwise Operator : simulink/Logic and Bit Operations/Bitwise Operator  logicop=AND  UseBitMask=on  BitMask=bin2dec('00000001')  BitMaskRealWorld=Stored Integer
  Bitwise Operator1 : simulink/Logic and Bit Operations/Bitwise Operator  logicop=AND  UseBitMask=on  BitMask=bin2dec('00000010')  BitMaskRealWorld=Stored Integer
  Bitwise Operator2 : simulink/Logic and Bit Operations/Bitwise Operator  logicop=AND  UseBitMask=on  BitMask=bin2dec('00000100')  BitMaskRealWorld=Stored Integer
  ChrgOvrCurrCntChk : Subsystem
  Compare To Constant : simulink/Logic and Bit Operations/Compare To Constant  relop===  const=1  OutDataTypeStr=boolean
  Compare To Constant1 : simulink/Logic and Bit Operations/Compare To Constant  relop===  const=2  OutDataTypeStr=boolean
  Compare To Constant2 : simulink/Logic and Bit Operations/Compare To Constant  relop===  const=4  OutDataTypeStr=boolean
  Constant : Constant  Value=boolean(0)  OutDataTypeStr=boolean
  Constant2 : Constant  Value=BSER_cntBattPrfDiag_CW
  Constant3 : Constant  Value=boolean(1)  OutDataTypeStr=boolean
  Constant4 : Constant  Value=boolean(0)  OutDataTypeStr=boolean
  Constant5 : Constant  Value=boolean(1)  OutDataTypeStr=boolean
  Constant6 : Constant  Value=boolean(0)  OutDataTypeStr=boolean
  Constant7 : Constant  Value=boolean(1)  OutDataTypeStr=boolean
  DSM_ReportCheck : Subsystem  TreatAsAtomicUnit=on  RTWFcnName=DSM_ReportCheck  RTWFileName=SrvLib
  DSM_ReportCheck1 : Subsystem  TreatAsAtomicUnit=on  RTWFcnName=DSM_ReportCheck  RTWFileName=SrvLib
  DSM_ReportCheck2 : Subsystem  TreatAsAtomicUnit=on  RTWFcnName=DSM_ReportCheck  RTWFileName=SrvLib
  Data Store Read : DataStoreRead  DataStoreName=DFC_ChrgOCNpl
  Data Store Read1 : DataStoreRead  DataStoreName=DFC_ChrgOCMax
  Data Store Read2 : DataStoreRead  DataStoreName=DFC_ChrgOCMin
  Data Store Write : DataStoreWrite  DataStoreName=DFC_ChrgOCNpl
  Data Store Write1 : DataStoreWrite  DataStoreName=DFC_ChrgOCMax
  Data Store Write2 : DataStoreWrite  DataStoreName=DFC_ChrgOCMin
  Switch{,1..5} (6 alike) : Switch  Criteria=u2 > Threshold
  BSER_bChrgOCNplDet : Outport
  BSER_bChrgOCNplHeal : Outport  Port=2
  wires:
  DSM_ReportCheck2/1(Dfc_id) -> Data Store Write/1
  Data Store Read/1 -> DSM_ReportCheck2/1(Dfc_id_nv)
  DSM_ReportCheck/1(Dfc_id) -> Data Store Write1/1
  Data Store Read1/1 -> DSM_ReportCheck/1(Dfc_id_nv)
  DSM_ReportCheck1/1(Dfc_id) -> Data Store Write2/1
  Data Store Read2/1 -> DSM_ReportCheck1/1(Dfc_id_nv)
  Constant/1 -> Switch/3
  Constant2/1 -> Bitwise Operator/1, Bitwise Operator2/1, Bitwise Operator1/1
  Switch/1 -> DSM_ReportCheck2/2(Err)
  Bitwise Operator/1 -> Compare To Constant/1
  Compare To Constant/1 -> Switch1/2, Switch/2
  Constant3/1 -> Switch1/3
  Switch1/1 -> DSM_ReportCheck2/3(Heal)
  Constant4/1 -> Switch2/3
  Compare To Constant1/1 -> Switch3/2, Switch2/2
  Bitwise Operator1/1 -> Compare To Constant1/1
  Constant5/1 -> Switch3/3
  BSER_bChrgOCMaxDet/1 -> Switch2/1
  Switch2/1 -> DSM_ReportCheck/2(Err), ChrgOvrCurrCntChk/1(BSER_bChrgOCMaxDet)
  BSER_bChrgOCMaxHeal/1 -> Switch3/1
  Switch3/1 -> DSM_ReportCheck/3(Heal)
  Constant6/1 -> Switch4/3
  Compare To Constant2/1 -> Switch5/2, Switch4/2
  Bitwise Operator2/1 -> Compare To Constant2/1
  Constant7/1 -> Switch5/3
  Switch4/1 -> DSM_ReportCheck1/2(Err), ChrgOvrCurrCntChk/2(BSER_bChrgOCMinDet)
  BSER_bChrgOCMinHeal/1 -> Switch5/1
  BSER_bChrgOCMinDet/1 -> Switch4/1
  Switch5/1 -> DSM_ReportCheck1/3(Heal)
  ChrgOvrCurrCntChk/2(BSER_bChrgOCNplDet) -> BSER_bChrgOCNplDet/1, Switch/1
  ChrgOvrCurrCntChk/1(BSER_bChrgOCNplHeal) -> Switch1/1, BSER_bChrgOCNplHeal/1

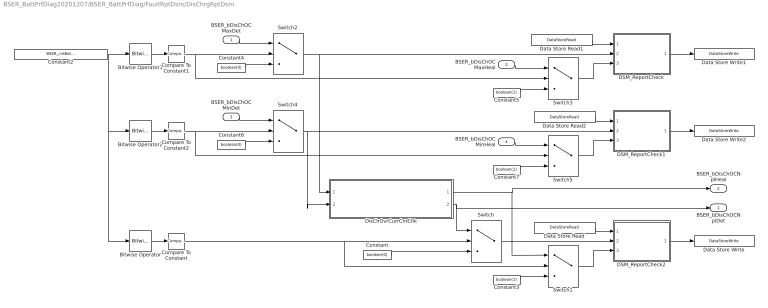
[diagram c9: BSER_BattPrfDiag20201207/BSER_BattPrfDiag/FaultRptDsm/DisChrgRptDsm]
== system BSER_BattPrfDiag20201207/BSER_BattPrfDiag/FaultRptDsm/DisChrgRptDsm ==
  BSER_bDisChOCMaxDet : Inport
  BSER_bDisChOCMaxHeal : Inport  Port=2
  BSER_bDisChOCMinDet : Inport  Port=3
  BSER_bDisChOCMinHeal : Inport  Port=4
  Bitwise Operator : simulink/Logic and Bit Operations/Bitwise Operator  logicop=AND  UseBitMask=on  BitMask=bin2dec('00001000')  BitMaskRealWorld=Stored Integer
  Bitwise Operator1 : simulink/Logic and Bit Operations/Bitwise Operator  logicop=AND  UseBitMask=on  BitMask=bin2dec('00010000')  BitMaskRealWorld=Stored Integer
  Bitwise Operator2 : simulink/Logic and Bit Operations/Bitwise Operator  logicop=AND  UseBitMask=on  BitMask=bin2dec('00100000')  BitMaskRealWorld=Stored Integer
  Compare To Constant : simulink/Logic and Bit Operations/Compare To Constant  relop===  const=8  OutDataTypeStr=boolean
  Compare To Constant1 : simulink/Logic and Bit Operations/Compare To Constant  relop===  const=16  OutDataTypeStr=boolean
  Compare To Constant2 : simulink/Logic and Bit Operations/Compare To Constant  relop===  const=32  OutDataTypeStr=boolean
  Constant : Constant  Value=boolean(0)  OutDataTypeStr=boolean
  Constant2 : Constant  Value=BSER_cntBattPrfDiag_CW
  Constant3 : Constant  Value=boolean(1)  OutDataTypeStr=boolean
  Constant4 : Constant  Value=boolean(0)  OutDataTypeStr=boolean
  Constant5 : Constant  Value=boolean(1)  OutDataTypeStr=boolean
  Constant6 : Constant  Value=boolean(0)  OutDataTypeStr=boolean
  Constant7 : Constant  Value=boolean(1)  OutDataTypeStr=boolean
  DSM_ReportCheck : Subsystem  TreatAsAtomicUnit=on  RTWFcnName=DSM_ReportCheck  RTWFileName=SrvLib
  DSM_ReportCheck1 : Subsystem  TreatAsAtomicUnit=on  RTWFcnName=DSM_ReportCheck  RTWFileName=SrvLib
  DSM_ReportCheck2 : Subsystem  TreatAsAtomicUnit=on  RTWFcnName=DSM_ReportCheck  RTWFileName=SrvLib
  Data Store Read : DataStoreRead  DataStoreName=DFC_DisChOCNpl
  Data Store Read1 : DataStoreRead  DataStoreName=DFC_DisChOCMax
  Data Store Read2 : DataStoreRead  DataStoreName=DFC_DisChOCMin
  Data Store Write : DataStoreWrite  DataStoreName=DFC_DisChOCNpl
  Data Store Write1 : DataStoreWrite  DataStoreName=DFC_DisChOCMax
  Data Store Write2 : DataStoreWrite  DataStoreName=DFC_DisChOCMin
  DisChOvrCurrCntChk : Subsystem
  Switch{,1..5} (6 alike) : Switch  Criteria=u2 > Threshold
  BSER_bDisChOCNplDet : Outport
  BSER_bDisChOCNplHeal : Outport  Port=2
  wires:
  DSM_ReportCheck2/1(Dfc_id) -> Data Store Write/1
  Data Store Read/1 -> DSM_ReportCheck2/1(Dfc_id_nv)
  DSM_ReportCheck/1(Dfc_id) -> Data Store Write1/1
  Data Store Read1/1 -> DSM_ReportCheck/1(Dfc_id_nv)
  DSM_ReportCheck1/1(Dfc_id) -> Data Store Write2/1
  Data Store Read2/1 -> DSM_ReportCheck1/1(Dfc_id_nv)
  Constant/1 -> Switch/3
  Constant2/1 -> Bitwise Operator/1, Bitwise Operator2/1, Bitwise Operator1/1
  DisChOvrCurrCntChk/2(BSER_bDisChOCNplDet) -> BSER_bDisChOCNplDet/1, Switch/1
  Switch/1 -> DSM_ReportCheck2/2(Err)
  Bitwise Operator/1 -> Compare To Constant/1
  Compare To Constant/1 -> Switch1/2, Switch/2
  Constant3/1 -> Switch1/3
  Switch1/1 -> DSM_ReportCheck2/3(Heal)
  DisChOvrCurrCntChk/1(BSER_bDisChOCNplHeal) -> BSER_bDisChOCNplHeal/1, Switch1/1
  Constant4/1 -> Switch2/3
  Compare To Constant1/1 -> Switch3/2, Switch2/2
  Bitwise Operator1/1 -> Compare To Constant1/1
  Constant5/1 -> Switch3/3
  BSER_bDisChOCMaxDet/1 -> Switch2/1
  Switch2/1 -> DSM_ReportCheck/2(Err), DisChOvrCurrCntChk/1(BSER_bDisChOCMaxDet)
  BSER_bDisChOCMaxHeal/1 -> Switch3/1
  Switch3/1 -> DSM_ReportCheck/3(Heal)
  Constant6/1 -> Switch4/3
  Compare To Constant2/1 -> Switch4/2, Switch5/2
  Bitwise Operator2/1 -> Compare To Constant2/1
  Constant7/1 -> Switch5/3
  Switch4/1 -> DSM_ReportCheck1/2(Err), DisChOvrCurrCntChk/2(BSER_bDisChOCMinDet)
  BSER_bDisChOCMinHeal/1 -> Switch5/1
  BSER_bDisChOCMinDet/1 -> Switch4/1
  Switch5/1 -> DSM_ReportCheck1/3(Heal)

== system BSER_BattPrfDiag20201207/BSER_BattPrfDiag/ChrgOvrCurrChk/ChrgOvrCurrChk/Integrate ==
  In : Inport
  Add : Sum
  Delay : Delay  DelayLength=1  InitialCondition=0
  Gain : Gain  Gain=0.01
  Saturation : Saturate  UpperLimit=15000  LowerLimit=0
  Out : Outport
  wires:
  Saturation/1 -> Delay/1, Out/1
  In/1 -> Gain/1
  Delay/1 -> Add/1
  Add/1 -> Saturation/1
  Gain/1 -> Add/2

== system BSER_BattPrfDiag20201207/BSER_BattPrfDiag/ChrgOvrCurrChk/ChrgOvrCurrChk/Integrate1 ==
  In : Inport
  Add : Sum
  Delay : Delay  DelayLength=1  InitialCondition=0
  Gain : Gain  Gain=0.01
  Saturation : Saturate  UpperLimit=30000  LowerLimit=0
  Out : Outport
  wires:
  Add/1 -> Saturation/1
  Delay/1 -> Add/1
  In/1 -> Gain/1
  Saturation/1 -> Out/1, Delay/1
  Gain/1 -> Add/2

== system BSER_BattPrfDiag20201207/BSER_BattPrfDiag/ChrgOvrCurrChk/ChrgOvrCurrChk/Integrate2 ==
  In : Inport
  Add : Sum
  Delay : Delay  DelayLength=1  InitialCondition=0
  Gain : Gain  Gain=0.01
  Saturation : Saturate  UpperLimit=15000  LowerLimit=0
  Out : Outport
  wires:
  Saturation/1 -> Delay/1, Out/1
  In/1 -> Gain/1
  Delay/1 -> Add/1
  Add/1 -> Saturation/1
  Gain/1 -> Add/2

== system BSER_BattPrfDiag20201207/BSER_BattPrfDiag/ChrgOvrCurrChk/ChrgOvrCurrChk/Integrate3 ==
  In : Inport
  Add : Sum
  Delay : Delay  DelayLength=1  InitialCondition=0
  Gain : Gain  Gain=0.01
  Saturation : Saturate  UpperLimit=30000  LowerLimit=0
  Out : Outport
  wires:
  Add/1 -> Saturation/1
  Delay/1 -> Add/1
  In/1 -> Gain/1
  Saturation/1 -> Out/1, Delay/1
  Gain/1 -> Add/2

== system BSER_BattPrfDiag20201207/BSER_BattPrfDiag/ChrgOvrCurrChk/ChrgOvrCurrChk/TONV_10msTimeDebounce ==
  note: Turn On Delay Time Deboune
  u : Inport
  T : Inport  Port=2
  Add : Sum
  Constant1 : Constant  Value=0  OutDataTypeStr=single
  Constant2 : Constant  OutDataTypeStr=uint8
  Constant3 : Constant  Value=0  OutDataTypeStr=uint8
  Constant4 : Constant  Value=0.01  OutDataTypeStr=single
  Delay : Delay  DelayLength=1  InitialCondition=0
  MinMax : MinMax  Inputs=2
  Product : Product  OutMin=[0]  OutMax=[65535]  OutDataTypeStr=single
  Relational Operator : RelationalOperator  Operator=>  OutDataTypeStr=boolean  RndMeth=Simplest
  Switch : Switch  Criteria=u2 ~= 0
  Switch1 : Switch  Criteria=u2 ~= 0
  y : Outport
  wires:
  MinMax/1 -> Add/2
  T/1 -> Relational Operator/2, MinMax/1
  Relational Operator/1 -> y/1
  Delay/1 -> MinMax/2
  Switch/1 -> Add/1
  Product/1 -> Delay/1, Relational Operator/1
  Add/1 -> Product/2
  Constant1/1 -> Switch/3
  Constant4/1 -> Switch/1
  u/1 -> Switch/2, Switch1/2
  Constant2/1 -> Switch1/1
  Constant3/1 -> Switch1/3
  Switch1/1 -> Product/1

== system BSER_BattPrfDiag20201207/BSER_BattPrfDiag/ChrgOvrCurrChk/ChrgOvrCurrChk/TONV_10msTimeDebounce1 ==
  note: Turn On Delay Time Deboune
  u : Inport
  T : Inport  Port=2
  Add : Sum
  Constant1 : Constant  Value=0  OutDataTypeStr=single
  Constant2 : Constant  OutDataTypeStr=uint8
  Constant3 : Constant  Value=0  OutDataTypeStr=uint8
  Constant4 : Constant  Value=0.01  OutDataTypeStr=single
  Delay : Delay  DelayLength=1  InitialCondition=0
  MinMax : MinMax  Inputs=2
  Product : Product  OutMin=[0]  OutMax=[65535]  OutDataTypeStr=single
  Relational Operator : RelationalOperator  Operator=>  OutDataTypeStr=boolean  RndMeth=Simplest
  Switch : Switch  Criteria=u2 ~= 0
  Switch1 : Switch  Criteria=u2 ~= 0
  y : Outport
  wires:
  Switch1/1 -> Product/1
  Constant3/1 -> Switch1/3
  Constant2/1 -> Switch1/1
  u/1 -> Switch1/2, Switch/2
  Constant4/1 -> Switch/1
  Constant1/1 -> Switch/3
  Add/1 -> Product/2
  Product/1 -> Relational Operator/1, Delay/1
  Switch/1 -> Add/1
  Delay/1 -> MinMax/2
  Relational Operator/1 -> y/1
  T/1 -> MinMax/1, Relational Operator/2
  MinMax/1 -> Add/2

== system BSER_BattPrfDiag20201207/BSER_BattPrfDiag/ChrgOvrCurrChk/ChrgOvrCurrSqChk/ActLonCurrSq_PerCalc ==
  BSPR_iCurr : Inport
  BSER_tiCurrConstPer_C : Inport  Port=2
  CurrProc : Stateflow chart  TreatAsAtomicUnit=on
  Sum of Elements : Sum  Inputs=+
  Terminator : Terminator
  Terminator1 : Terminator
  BSER_iCurrPerAcm : Outport
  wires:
  BSER_tiCurrConstPer_C/1 -> CurrProc/2(BSER_tiCurrCalcPer_C)
  Sum of Elements/1 -> BSER_iCurrPerAcm/1
  BSPR_iCurr/1 -> CurrProc/1(BSPR_iCurr)
  CurrProc/1(BSER_iCurrSqAvrgS_A) -> Sum of Elements/1
  CurrProc/3(i) -> Terminator1/1
  CurrProc/2(Index_s) -> Terminator/1
